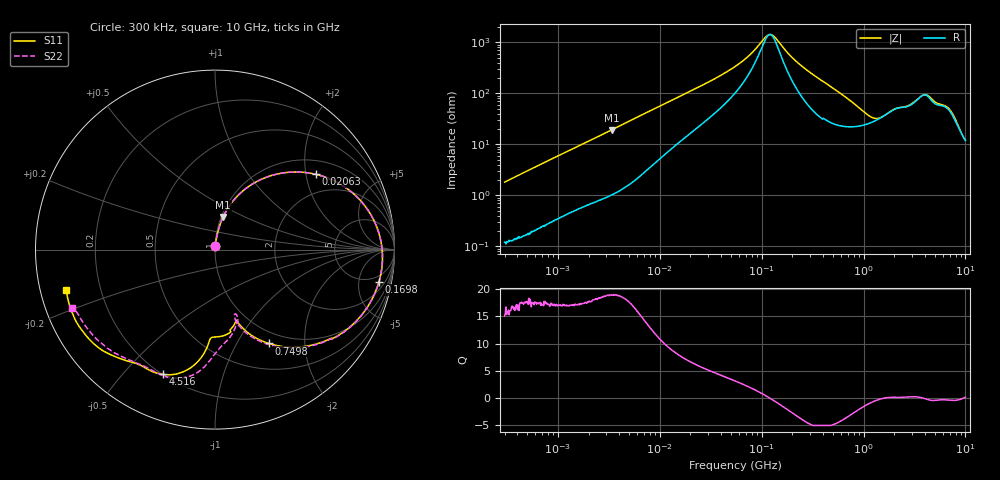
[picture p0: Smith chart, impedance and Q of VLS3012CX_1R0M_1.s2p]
! S-Parameter Data Generated by TDK Corporation
! Copyright(C) 2019 TDK Corporation.
! All Rights Reserved.
! TDK P/N: VLS3012CX-1R0M-1 (Inductor)
! Property: L=1uH at 1MHz
! Size(LxWxT): 3x3x1.2mm
! Model Type: s2p (Touchstone File Format Version 1.0)
! Frequency: DC=Yes Start=0.3MHz Stop=10000MHz 802points Log-sweep
! Model Generated on Sep. 23, 2019
! Port Assignments:
!  1 ---@@@--- 2
! Applicable Conditions:
!  Temperature = 25 degC
!  DC Bias Current = 0 A
!  Small Signal Operation
! Terms and conditions regarding TDK Simulation Models
! (1)This simulation model is being provided solely for informational purposes. Please refer to the specifications of the products in terms of detailed characteristics of such products.
! (2)In no event shall TDK Corporation of any of its subsidiaries be liable for any loss or damage arising, directly or indirectly,
!  From any information contained in this simulation model, including, but not limited to loss or damages arising from any inaccuracies, omissions or errors in connection with such information.
! (3)Any and all copyrights on this simulation model are owned by TDK Corporation.
!  Duplication or redistribution of this simulation model without prior written permission from TDK Corporation is prohibited.
! (4)This simulation model is subject to any modification or change without any prior notice.
! (5)Neither TDK Corporation nor any of its subsidiaries shall make any warranty, express or implied,
!  Including but not limited to the correctness, implied warranties of merchantability and fitness for a particular purpose with respect to this simulation models.
! (6)The use of this simulation model shall be deemed to have consented to the terms and conditions hereof.
# Hz S MA R 50
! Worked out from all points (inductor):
!   801 points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, 300 kHz to 10 GHz, reference 50 ohm
!   read as one part in series: L = 961 nH near 318.3 kHz
!   highest Q = 18.9 at 3.375 MHz (marker M1), where L = 906 nH
!   self-resonance near 120.4 MHz
!   S11 on the Smith chart (normalised r, x): 300 kHz: 1.00, +0.04; 20.63 MHz: 1.38, +2.27; 169.8 MHz: 3.32, -8.99; 749.8 MHz: 0.83, -1.37; 4.516 GHz: 0.20, -0.65; 10 GHz: 0.08, -0.13
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300000  0.01799 84.8  0.9985 -1.1  0.9988 -1.0  0.01793 85.5
1713600  0.09809 81.0  0.9895 -5.7  0.9894 -5.7  0.09808 81.0
3374880  0.1865 76.1  0.9726 -10.8  0.9726 -10.8  0.1864 76.1
5955893  0.3134 68.0  0.9301 -18.4  0.9301 -18.4  0.3134 68.0
9671944  0.4606 57.3  0.8471 -27.6  0.8472 -27.6  0.4606 57.3
2.063197e7  0.7 36.9  0.6152 -44.4  0.6152 -44.4  0.7 36.8
5.477226e7  0.8873 13.1  0.2654 -59.3  0.2654 -59.3  0.8872 13.1
7.329659e7  0.9135 7.0  0.174 -57.8  0.174 -57.8  0.9134 7.0
1.177683e8  0.9344 -2.8  0.06596 -9.0  0.06598 -9.0  0.9343 -2.9
1.323997e8  0.9354 -5.4  0.07117 20.1  0.0712 20.1  0.9353 -5.5
1.69821e8  0.9309 -11.2  0.1298 49.9  0.1298 49.9  0.9307 -11.4
3.126428e8  0.8728 -28.7  0.3488 50.1  0.3488 50.1  0.8723 -29.1
4.986356e8  0.7534 -45.1  0.5311 34.0  0.5311 34.0  0.752 -45.8
7.497801e8  0.6021 -60.3  0.6603 14.8  0.6603 14.8  0.5973 -61.4
1.165098e9  0.4476 -71.4  0.713 -9.5  0.713 -9.5  0.4297 -73.2
1.767019e9  0.4274 -75.2  0.6346 -34.5  0.6346 -34.5  0.3892 -71.5
2.798208e9  0.4932 -92.6  0.4993 -57.3  0.4991 -57.3  0.5513 -87.5
3.472057e9  0.5872 -96.3  0.383 -70.3  0.3827 -70.3  0.6493 -94.7
4.516006e9  0.753 -112.6  0.2878 -64.3  0.288 -64.2  0.7572 -110.0
7.06055e9  0.8293 -135.6  0.2425 -81.6  0.2423 -81.7  0.8092 -136.5
8.993752e9  0.8704 -154.5  0.226 -89.1  0.2255 -89.1  0.8458 -155.8
1e10  0.8581 -164.8  0.2251 -93.9  0.2248 -93.9  0.858 -157.8
